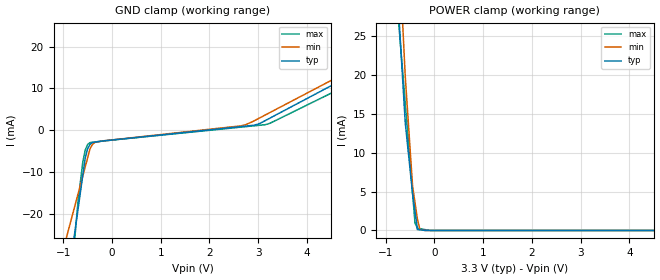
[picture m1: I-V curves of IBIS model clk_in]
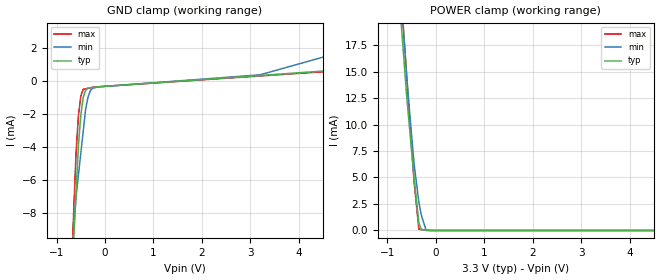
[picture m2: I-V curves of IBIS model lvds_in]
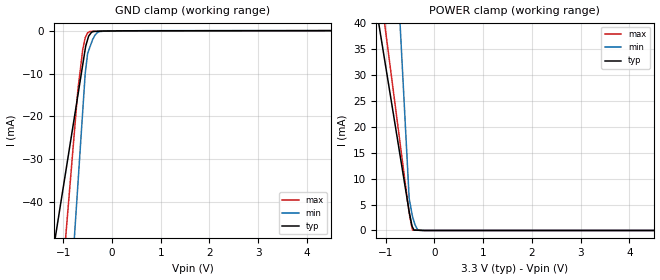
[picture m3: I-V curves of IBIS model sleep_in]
| Teraspeed (R) Labs.
| http://www.teraspeed.com
[IBIS Ver]   3.2
[Comment Char] |_char
[File Name]   dac5675amhfg.ibs
[File Rev]   B
[Date]   07-19-2011
[Notes]   Quality Check of this IBIS model: Model Passes IBIS Check
   Model parses into ICX IS. Simulation done with Hyperlynx.
   1. MIN TYP MAX information is based on Temprature and Voltage
   characteristics only.
   2. Package information extracted using Tektronix IConnect Software.
|04-14-2015  Modified for ceramic HFG package.   WVB
|10-08-2015  Modified order for CLK/CLK to comply with IBIS4.0
|   non-complementary pin must be listed first  WVB
|05-23-2016  Corrected differential pin ordering.   WVB
|   Pins CLK/CLKC, D6A/D6B, D7A/D7B
|   Removed CLK/CLKC from series mapping.
[Disclaimer]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
[Source]
| This model file was created by Teraspeed Consulting Group LLC
| (http://www.teraspeed.com/).
[Disclaimer]
| This product is designed as an aid for customers of Texas Instruments.
| No warranties, either expressed or implied, with respect to this third
| party software (if any) or with respect to its fitness for any
| particular purpose is claimed by Texas Instruments or the author. The
| software (if any) is provided solely on an "as is" basis. The entire
| risk as to its quality and performance is with the customer
[Copyright]
| (C) Copyright 2011 Texas Instruments Incorporated. All rights reserved.
| All other rights are reserved.
[Component]   DAC5675AMHFG
[Manufacturer] TI
[Package]
| variable   typ   min   max
R_pkg  2.920E-01  2.720E-01  3.100E-01
L_pkg  4.015E-09  2.812E-09  5.086E-09
C_pkg  1.071E-12  9.160E-13  1.204E-12
[Pin] signal_name  model_name  R_pin  L_pin C_pin
1   D13A   lvds_in  3.100E-01   5.086E-09   1.204E-12
2   D13B   lvds_in  3.040E-01   4.687E-09   1.156E-12
3   D12A   lvds_in  2.960E-01   4.296E-09   1.108E-12
4   D12B   lvds_in  2.900E-01   3.913E-09   1.060E-12
5   D11A   lvds_in  2.840E-01   3.538E-09   1.012E-12
6   D11B   lvds_in  2.780E-01   3.171E-09   9.640E-13
7   D10A   lvds_in  2.720E-01   2.812E-09   9.160E-13
8   D10B   lvds_in  2.780E-01   3.171E-09   9.640E-13
9   D9A   lvds_in  2.840E-01   3.538E-09   1.012E-12
10  D9B   lvds_in  2.900E-01   3.913E-09   1.060E-12
11  D8A   lvds_in  2.960E-01   4.296E-09   1.108E-12
12  D8B   lvds_in  3.040E-01   4.687E-09   1.156E-12
13  AGND   GND   3.100E-01   5.086E-09   1.204E-12
14  D7A   lvds_in  3.100E-01   5.086E-09   1.204E-12
15  D7B   lvds_in  3.040E-01   4.687E-09   1.156E-12
16  DVDD   POWER   2.960E-01   4.296E-09   1.108E-12
17  DGND   GND   2.900E-01   3.913E-09   1.060E-12
18  DVDD   POWER   2.840E-01   3.538E-09   1.012E-12
19  DGND   GND   2.780E-01   3.171E-09   9.640E-13
20  AGND   GND   2.720E-01   2.812E-09   9.160E-13
21  AVDD   POWER   2.780E-01   3.171E-09   9.640E-13
23  CLK   clk_in   2.900E-01   3.913E-09   1.060E-12
22  CLKC   clk_in   2.840E-01   3.538E-09   1.012E-12
24  D6A   lvds_in  2.960E-01   4.296E-09   1.108E-12
25  D6B   lvds_in  3.040E-01   4.687E-09   1.156E-12
26  AGND   GND   3.100E-01   5.086E-09   1.204E-12
27  D5A   lvds_in  3.100E-01   5.086E-09   1.204E-12
28  D5B   lvds_in  3.040E-01   4.687E-09   1.156E-12
29  D4A   lvds_in  2.960E-01   4.296E-09   1.108E-12
30  D4B   lvds_in  2.900E-01   3.913E-09   1.060E-12
31  D3A   lvds_in  2.840E-01   3.538E-09   1.012E-12
32  D3B   lvds_in  2.780E-01   3.171E-09   9.640E-13
33  D2A   lvds_in  2.720E-01   2.812E-09   9.160E-13
34  D2B   lvds_in  2.780E-01   3.171E-09   9.640E-13
35  D1A   lvds_in  2.840E-01   3.538E-09   1.012E-12
36  D1B   lvds_in  2.900E-01   3.913E-09   1.060E-12
37  D0A   lvds_in  2.960E-01   4.296E-09   1.108E-12
38  D0B   lvds_in  3.040E-01   4.687E-09   1.156E-12
39  AGND   GND   3.100E-01   5.086E-09   1.204E-12
40  SLEEP   sleep_in 3.100E-01   5.086E-09   1.204E-12
41  NC   NC   3.040E-01   4.687E-09   1.156E-12
42  BIASJ   term   2.960E-01   4.296E-09   1.108E-12
43  EXTIO   term   2.900E-01   3.913E-09   1.060E-12
44  AGND   GND   2.840E-01   3.538E-09   1.012E-12
45  AVDD   POWER   2.780E-01   3.171E-09   9.640E-13
46  IOUT1   analog   2.720E-01   2.812E-09   9.160E-13
47  IOUT2   analog   2.780E-01   3.171E-09   9.640E-13
48  AVDD   POWER   2.840E-01   3.538E-09   1.012E-12
49  AGND   GND   2.900E-01   3.913E-09   1.060E-12
50  AGND   GND   2.960E-01   4.296E-09   1.108E-12
51  AVDD   POWER   3.040E-01   4.687E-09   1.156E-12
52  AGND   GND   3.100E-01   5.086E-09   1.204E-12
[diff pin] inv_pin vdiff tdelay_typ tdelay_min tdelay_max
1   2  100mV  NA  NA  NA
3   4  100mV  NA  NA  NA
5   6  100mV  NA  NA  NA
7   8  100mV  NA  NA  NA
9   10  100mV  NA  NA  NA
11  12  100mV  NA  NA  NA
14  15  100mV  NA  NA  NA
23  22  400mV  NA  NA  NA
24  25  100mV  NA  NA  NA
27  28  100mV  NA  NA  NA
29  30  100mV  NA  NA  NA
31  32  100mV  NA  NA  NA
33  34  100mV  NA  NA  NA
35  36  100mV  NA  NA  NA
37  38  100mV  NA  NA  NA
[Series Pin Mapping]  pin_2  model_name
1   2  110ohm
3   4  110ohm
5   6  110ohm
7   8  110ohm
9   10  110ohm
11  12  110ohm
14  15  110ohm
24  25  110ohm
27  28  110ohm
29  30  110ohm
31  32  110ohm
33  34  110ohm
35  36  110ohm
37  38  110ohm
[Model] 110ohm
Model_type Series
| variable   typ   min   max
C_comp   0.00000pF 0.00000pF 0.00000pF
[Voltage Range] 3.30000V 3.15000V 3.45000V
[R Series] 110  90  132
[Model] analog
Model_type Terminator
C_comp  0.00000pF 0.00000pF 0.00000pF
| variable   typ   min   max
[Voltage Range]   3.3000V  3.1500V  3.4500V
[POWER Clamp Reference]  3.3000V  3.1500V  3.4500V
[GND Clamp Reference]   0.0000V  0.0000V  0.0000V
[Temperature Range]   25   125   -55
[Model] term
Model_type Terminator
C_comp  0.00000pF 0.00000pF 0.00000pF
| variable   typ   min   max
[Voltage Range]   3.3000V  3.1500V  3.4500V
[POWER Clamp Reference]  3.3000V  3.1500V  3.4500V
[GND Clamp Reference]   0.0000V  0.0000V  0.0000V
[Temperature Range]   25   125   -55
| Models and submodels in the file (6): 110ohm (Series), analog (Terminator), clk_in (Input), lvds_in (Input), sleep_in (Input), term (Terminator)
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[Model] clk_in
Model_type Input
Vinl = 1.60000V
Vinh = 2.40000V
C_comp 2.00000pF 2.00000pF 2.00000pF
| variable typ   min   max
[Voltage Range] 3.30000V 3.15000V 3.45000V
[POWER Clamp Reference] 3.30000V 3.15000V 3.45000V
[GND Clamp Reference] 0.00000V 0.00000V 0.00000V
[Temperature Range]   25   125   -55
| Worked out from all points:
|   POWER clamp passes 1 mA (typ) near -0.37 V on its own axis
[GND Clamp]
-3.3V     -235.6mA   -129.6mA   -365.3mA
-700mV    -19.2mA    -15.43mA   -17.4mA
-600mV    -10.88mA   -11.04mA   -7.717mA
-550mV    -6.717mA   -8.845mA   -4.83mA
-500mV    -4.508mA   -6.651mA   -3.457mA
-450mV    -3.391mA   -4.456mA   -3.007mA
-350mV    -2.892mA   -2.948mA   -2.854mA
-175mV    -2.606mA   -2.578mA   -2.605mA
2.65V     831.8uA    1.01mA     703.4uA
3V        1.422mA    2.714mA    1.113mA
3.25V     2.907mA    4.243mA    1.664mA
6.6V      23.58mA    24.73mA    20.89mA
[POWER Clamp]
-3.3V     296.9mA    367.3mA    224.2mA
-600mV    13.87mA    19.81mA    16.36mA
-450mV    4.767mA    5.737mA    4.815mA
-400mV    2.442mA    3.586mA    966uA
-350mV    117.3uA    1.434mA    290uA
-300mV    83.81uA    144.2uA    232uA
-200mV    16.76uA    0A         116uA
-75mV     0A         0A         0A
6.6V      0A         0A         0A
[Model] lvds_in
Model_type Input
Vinl = 1100.00mV
Vinh = 1.3000V
C_comp 2.00000pF 2.00000pF 2.00000pF
| variable typ   min   max
[Voltage Range] 3.30000V 3.15000V 3.45000V
[POWER Clamp Reference] 3.30000V 3.15000V 3.45000V
[GND Clamp Reference] 0.00000V 0.00000V 0.00000V
[Temperature Range]   25   125   -55
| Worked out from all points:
|   GND clamp passes 1 mA (typ) near -0.45 V on its own axis
|   POWER clamp passes 1 mA (typ) near -0.36 V on its own axis
[GND Clamp]
-3.3V     -164.4mA   -124.7mA   -204.6mA
-600mV    -6.813mA   -7.033mA   -4.418mA
-550mV    -3.894mA   -5.7mA     -2.115mA
-500mV    -2.059mA   -4.367mA   -909.1uA
-450mV    -993.7uA   -3.034mA   -502.3uA
-400mV    -558.2uA   -1.701mA   -472.1uA
-350mV    -428.5uA   -951.4uA   -441.8uA
-300mV    -409.1uA   -580.5uA   -411.6uA
-250mV    -389.8uA   -435.3uA   -381.4uA
-125mV    -350.5uA   -353.8uA   -346.8uA
3.2V      329.9uA    370.1uA    300.6uA
6.6V      1.026mA    3.158mA    962.6uA
[POWER Clamp]
-3.3V     176.5mA    194.6mA    191.7mA
-600mV    12.58mA    14.34mA    14.51mA
-450mV    5.01mA     6.33mA     4.67mA
-350mV    695uA      2.654mA    108.7uA
-300mV    102.3uA    1.461mA    86.96uA
-200mV    34.09uA    0A         43.48uA
6.6V      0A         0A         0A
[Model] sleep_in
Model_type Input
Vinl = 800.000mV
Vinh = 2.00000V
C_comp 2.00000pF 2.00000pF 2.00000pF
| variable typ   min   max
[Voltage Range] 3.30000V 3.15000V 3.45000V
[POWER Clamp Reference] 3.30000V 3.15000V 3.45000V
[GND Clamp Reference] 0.00000V 0.00000V 0.00000V
[Temperature Range]   25   125   -55
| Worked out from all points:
|   GND clamp passes 1 mA (typ) near -0.47 V on its own axis
|   POWER clamp passes 1 mA (typ) near -0.46 V on its own axis
[GND Clamp]
-3.3V     -201.7mA   -485.5mA   -371.5mA
-700mV    -15.05mA   -35.93mA   -13.79mA
-600mV    -7.869mA   -18.63mA   -4.318mA
-550mV    -4.279mA   -9.988mA   -1.613mA
-540mV    -3.561mA   -9.043mA   -1.378mA
-500mV    -2.006mA   -5.265mA   -435.6uA
-480mV    -1.228mA   -4.628mA   -308.6uA
-450mV    -766.9uA   -3.673mA   -118.2uA
-400mV    -214.7uA   -2.081mA   -100.5uA
-300mV    -86.34uA   -392.9uA   -65.18uA
-125mV    -25.47uA   -20.9uA    -23.48uA
6.6V      82.28uA    83.68uA    70.72uA
[POWER Clamp]
-3.3V     165mA      507.1mA    205mA
-650mV    11.19mA    29.61mA    12.75mA
-520mV    3.643mA    6.191mA    3.316mA
-460mV    797.3uA    3.102mA    420.8uA
-450mV    618.1uA    2.662mA    59.81uA
-420mV    80.18uA    1.724mA    53.83uA
-400mV    72.55uA    1.099mA    49.84uA
-350mV    53.45uA    182.4uA    39.87uA
-250mV    15.27uA    12.34uA    19.94uA
6.6V      0A         0A         0A
